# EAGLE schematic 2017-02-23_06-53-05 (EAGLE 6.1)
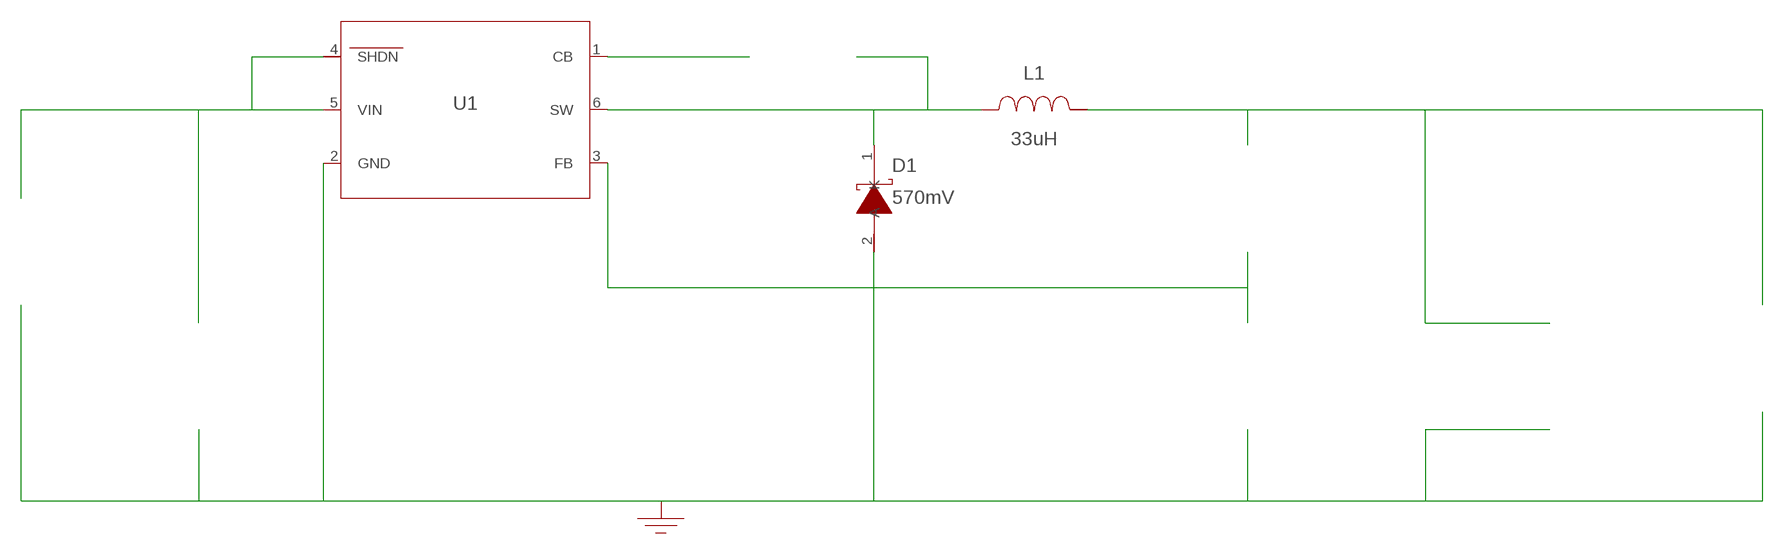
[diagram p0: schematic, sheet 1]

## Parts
CBOOT  150nF  GRM155R60J154KE01DGRM155R60J154KE01D  [0402]  (not placed on a sheet)
CIN  1uF  C1608X5R1H105K080ABC1608X5R1H105K080AB  [0603]  (not placed on a sheet)
COUT  22uF  GRM21BR60J226ME39LGRM21BR60J226ME39L  [0805]  (not placed on a sheet)
COUT_2  22uF  GRM21BR60J226ME39LGRM21BR60J226ME39L  [0805]  (not placed on a sheet)
D1  570mV  PMEG6010CEH,115PMEG6010CEH,115  [SOD-123F]
GND  WB_GND  WB_GNDWB_GND  [WB_GND]
IOUT  WB_CURRENT_LOAD  WB_CURRENT_LOADWB_CURRENT_LOAD  [WB_CURRENT_LOAD]  (not placed on a sheet)
L1  33uH  SRN6045-330MSRN6045-330M  [SRN6045]
RFB1  1k  CRCW04021K00FKEDCRCW04021K00FKED  [0402]  (not placed on a sheet)
RFB2  5.49k  CRCW04025K49FKEDCRCW04025K49FKED  [0402]  (not placed on a sheet)
U1  LMR14206XMKE/NOPB  LMR14206XMKE/NOPBLMR14206XMKE/NOPB  [MK06A]
VIN  WB_BATTERY  WB_BATTERYWB_BATTERY  [WB_BATTERY]  (not placed on a sheet)

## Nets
0: Cin.2@2 Cout.2@2 Cout_2.2@2 D1.2(A) GND.1 Iout.-@2 Rfb1.1@1 U1.2(GND) Vin.-@2
1: Cin.1@1 U1.4(SHDN) U1.5(VIN) Vin.+@1
2: Rfb1.2@2 Rfb2.1@1 U1.3(FB)
3: Cboot.1@1 D1.1(K) L1.1 U1.6(SW)
4: Cboot.2@2 U1.1(CB)
5: Cout.1@1 Cout_2.1@1 Iout.+@1 L1.2 Rfb2.2@2
Unconnected: CBOOT.1 CBOOT.2 CIN.1 CIN.2 COUT.1 COUT.2 COUT_2.1 COUT_2.2 IOUT.1(+) IOUT.2(-) RFB1.1 RFB1.2 RFB2.1 RFB2.2 VIN.1(+) VIN.2(-)

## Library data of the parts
CBOOT = AcceleratedDesigns_Lib:GRM155R60J154KE01D; Cap: 1.5E-7; ESR: 0.0; IRMS: 0.0; Manufacturer_Name: MuRata; Manufacturer_Part_Number: GRM155R60J154KE01D; VDC: 6.3; Vendor: MuRata
CIN = AcceleratedDesigns_Lib:C1608X5R1H105K080AB; Cap: 1.0E-6; Datasheet_URL: https://product.tdk.com/en/search/capacitor/ceramic/mlcc/info?part%5Fno%3DC1608X5R1H105K080AB; ESR: 0.005522; IRMS: 2.21617; Manufacturer_Name: TDK; Manufacturer_Part_Number: C1608X5R1H105K080AB; VDC: 50.0; Vendor: TDK
COUT COUT_2 = AcceleratedDesigns_Lib:GRM21BR60J226ME39L; Cap: 2.2E-5; ESR: 0.0; IRMS: 0.0; Manufacturer_Name: MuRata; Manufacturer_Part_Number: GRM21BR60J226ME39L; VDC: 6.3; Vendor: MuRata
D1 = AcceleratedDesigns_Lib:PMEG6010CEH,115; Datasheet_URL: http://www.nxp.com/documents/data%5Fsheet/PMEG6010CEH%5FPMEG6010CEJ.pdf; Io: 1.0; Manufacturer_Name: NXP Semiconductor; Manufacturer_Part_Number: PMEG6010CEH,115; VFatIo: 0.57; VRRM: 60.0; Vendor: NXP Semiconductor
GND = AcceleratedDesigns_Lib:WB_GND; Manufacturer_Name: WB_GND; Manufacturer_Part_Number: WB_GND; PowerPortType: POWER_GROUND; Value: Value
IOUT = AcceleratedDesigns_Lib:WB_CURRENT_LOAD; Manufacturer_Name: WB_CURRENT_LOAD; Manufacturer_Part_Number: WB_CURRENT_LOAD; PowerPortType: POWER_GROUND; Value: Value
L1 = AcceleratedDesigns_Lib:SRN6045-330M; DCR: 0.188; Datasheet_URL: http://www.bourns.com/data/global/pdfs/SRN6045.pdf; IDC: 1.4; L: 3.3E-5; Manufacturer_Name: Bourns; Manufacturer_Part_Number: SRN6045-330M; Vendor: Bourns
RFB1 = AcceleratedDesigns_Lib:CRCW04021K00FKED; Manufacturer_Name: Vishay-Dale; Manufacturer_Part_Number: CRCW04021K00FKED; Power: 0.063; Resistance: 1000.0; Tolerance: 1.0; Vendor: Vishay-Dale
RFB2 = AcceleratedDesigns_Lib:CRCW04025K49FKED; Manufacturer_Name: Vishay-Dale; Manufacturer_Part_Number: CRCW04025K49FKED; Power: 0.063; Resistance: 5490.0; Tolerance: 1.0; Vendor: Vishay-Dale
U1 = AcceleratedDesigns_Lib:LMR14206XMKE/NOPB; Datasheet_URL: http://www.ti.com/product/lmr14206x; Frequency: 1200000.0; Imax: 0.6; Manufacturer_Name: Texas Instruments; Manufacturer_Part_Number: LMR14206XMK/NOPB; Mktg_Package: NA; NSID: LMR14206XMK/NOPB; Package: NA; Vendor: Texas Instruments
VIN = AcceleratedDesigns_Lib:WB_BATTERY; Manufacturer_Name: WB_BATTERY; Manufacturer_Part_Number: WB_BATTERY; PowerPortType: POWER_GROUND; Value: Value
